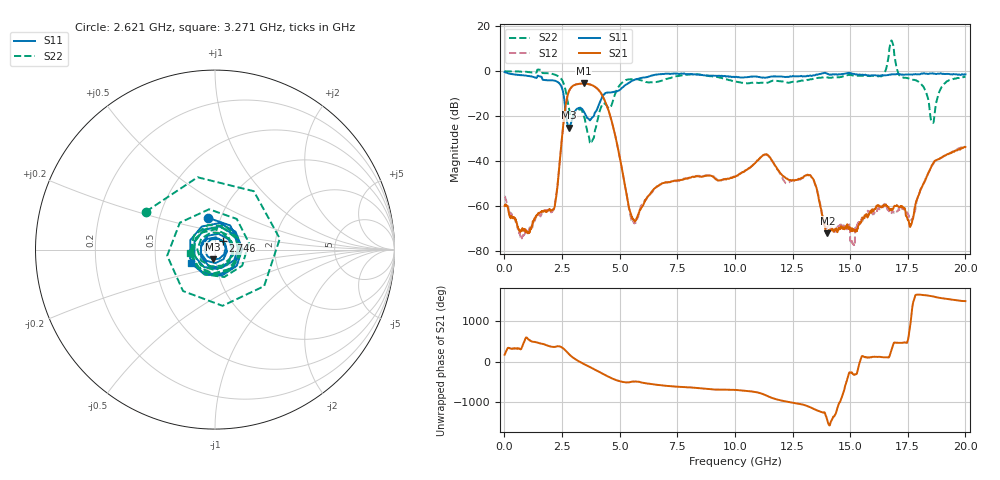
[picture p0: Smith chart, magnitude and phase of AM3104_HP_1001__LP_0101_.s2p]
!Created with skrf (http://scikit-rf.org).
# Hz S RI R 50.0
!freq ReS11 ImS11 ReS21 ImS21 ReS12 ImS12 ReS22 ImS22
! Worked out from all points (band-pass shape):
!   1601 points, 10 MHz to 20 GHz, reference 50 ohm
!   highest |S21| = -5.48 dB at 3.433 GHz (marker M1); lowest = -72.1 dB at 14.02 GHz (marker M2)
!   |S21| within 3 dB of the highest: 2.821 GHz to 4.099 GHz (1.278 GHz wide, 36.9 % of centre)
!   lowest |S11| = -25.1 dB at 2.796 GHz (marker M3), VSWR 1.12, Z = 48.6 - j5.33 ohm
!   |S11| at or under -10 dB: 2.561 GHz to 4.355 GHz (1.793 GHz wide, 51.9 % of centre)
!   |S22| runs from -31.7 to 13.6 dB; largest |S21 - S12| = 0.026
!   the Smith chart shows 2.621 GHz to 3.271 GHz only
!   S11 on the Smith chart (normalised r, x): 2.621 GHz: 0.87, +0.32; 2.746 GHz: 1.08, +0.10; 3.271 GHz: 0.76, -0.12
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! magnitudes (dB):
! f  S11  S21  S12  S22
! 10 MHz  -0.4  -59.8  -55.7  -0.1
! 772.1 MHz  -1.8  -70.5  -73.4  -0.2
! 2.084 GHz  -4.1  -61.7  -62.3  -1.2
! 2.621 GHz  -14.8  -18.0  -18.0  -7.2
! 2.746 GHz  -23.9  -10.7  -10.7  -13.6
! 2.796 GHz  -25.1  -9.1  -9.1  -16.5
! 3.271 GHz  -16.3  -5.6  -5.7  -17.0
! 3.346 GHz  -16.6  -5.5  -5.6  -17.2
! 3.433 GHz  -17.8  -5.5  -5.5  -19.8
! 3.783 GHz  -20.9  -6.2  -6.2  -31.2
! 4.445 GHz  -9.5  -15.3  -15.3  -15.4
! 5.57 GHz  -4.2  -65.7  -66.6  -3.6
! 6.682 GHz  -1.4  -50.9  -51.0  -4.6
! 10.01 GHz  -2.7  -47.0  -46.9  -4.6
! 11.33 GHz  -2.9  -37.0  -37.3  -5.1
! 13.34 GHz  -2.1  -47.2  -47.2  -3.6
! 14.02 GHz  -1.2  -72.1  -69.4  -2.8
! 15.1 GHz  -1.2  -70.5  -76.3  -1.9
! 16.68 GHz  -1.6  -60.9  -62.2  7.2
! 17.64 GHz  -1.4  -67.9  -65.4  -3.6
! 18.56 GHz  -0.9  -41.4  -41.8  -22.7
! 20 GHz  -1.4  -33.7  -33.2  -2.5
